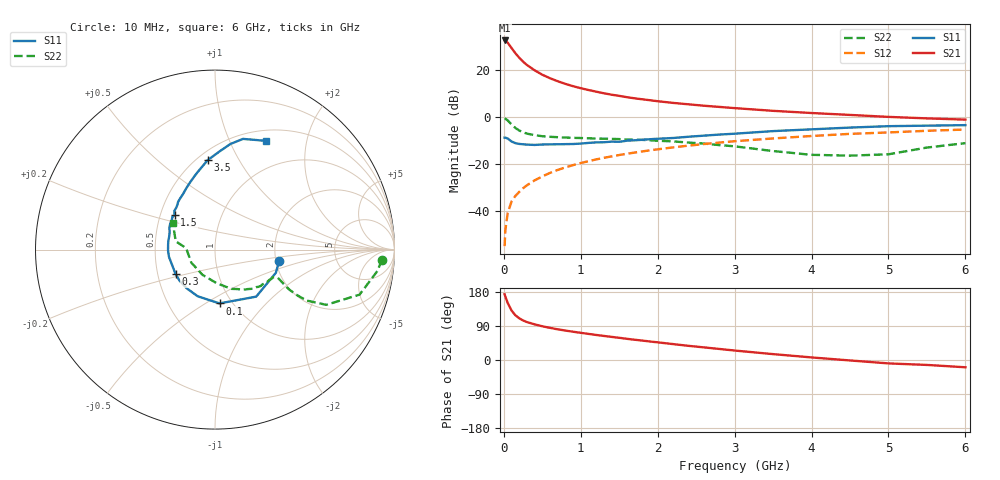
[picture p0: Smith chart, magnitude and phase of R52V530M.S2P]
! SIEMENS Small Signal Semiconductors
! BFR183
! Si NPN RF Bipolar Junction Transistor in SOT23
! VCE = 2.5 V  IC = 30 mA
! Common Emitter S-Parameters:  May  1996
# GHz  S  MA  R  50
!  f  S11  S21  S12  S22
! GHz  MAG  ANG  MAG  ANG  MAG  ANG  MAG  ANG
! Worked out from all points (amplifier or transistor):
!   36 points, 10 MHz to 6 GHz, reference 50 ohm
!   highest |S21| = 32.5 dB at 10 MHz (marker M1)
!   |S21| within 3 dB of that: start of sweep to 95.48 MHz
!   unconditionally stable (mu >= 1): 394.8 MHz to 2.371 GHz
!   at 250 MHz: K = 0.91, MSG = 26.9 dB, |S12| = -30.3 dB
!   at 1.4 GHz: K = 1.05, MAG = 11.7 dB, |S12| = -16.8 dB
!   at 6 GHz: K = 0.91, MSG = 2.1 dB, |S12| = -5.4 dB
!   S11 on the Smith chart (normalised r, x): 10 MHz: 2.08, -0.32; 100 MHz: 0.87, -0.58; 300 MHz: 0.62, -0.18; 1.5 GHz: 0.59, +0.25; 3.5 GHz: 0.56, +0.75; 6 GHz: 0.63, +1.38
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0.01  0.363 -10.5  42.07 173.5  0.0018 87.1  0.9319 -3.4
0.02  0.3628 -20.9  41.5 167.1  0.004 79.8  0.9128 -7.5
0.05  0.3483 -48.8  37.61 150.6  0.0091 75.1  0.8436 -17.3
0.1  0.3008 -85.2  29.1 130.8  0.016 71.6  0.6921 -26.4
0.15  0.2774 -110.4  22.53 118.0  0.021 69.5  0.5827 -29.1
0.2  0.267 -126.2  18.07 110.1  0.0255 71.2  0.5151 -29.0
0.25  0.2626 -139.0  14.91 104.4  0.0305 71.3  0.4702 -28.3
0.3  0.2584 -148.3  12.69 100.1  0.0353 72.2  0.4427 -27.3
0.4  0.2542 -161.8  9.779 94.1  0.0449 73.5  0.4093 -25.6
0.5  0.2596 -171.1  7.87 89.0  0.0545 74.2  0.3893 -24.5
0.6  0.2617 -178.8  6.628 84.8  0.0648 73.9  0.3785 -24.3
0.7  0.2626 174.3  5.733 81.0  0.0748 73.5  0.3712 -24.5
0.8  0.2644 169.5  5.031 77.7  0.0847 72.9  0.3646 -24.9
0.9  0.2659 163.4  4.494 74.6  0.0948 72.3  0.3596 -25.4
1.1  0.2807 155.1  3.73 68.9  0.1148 70.8  0.3522 -27.9
1.5  0.2962 139.6  2.798 58.6  0.1552 66.9  0.3381 -33.4
1.7  0.319 132.3  2.484 53.5  0.1749 64.7  0.3277 -36.3
2.2  0.3569 120.0  1.985 42.0  0.2254 58.8  0.3021 -46.2
3.5  0.5 94.7  1.347 15.5  0.3491 41.7  0.1884 -86.8
4.5  0.5939 81.8  1.103 -1.2  0.4368 28.6  0.1507 -151.0
5.5  0.6523 69.4  0.931 -13.0  0.5076 16.5  0.2237 168.0
6  0.6693 64.7  0.877 -19.2  0.5397 8.8  0.2772 147.9
